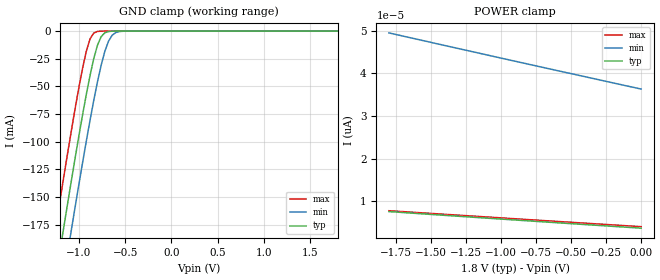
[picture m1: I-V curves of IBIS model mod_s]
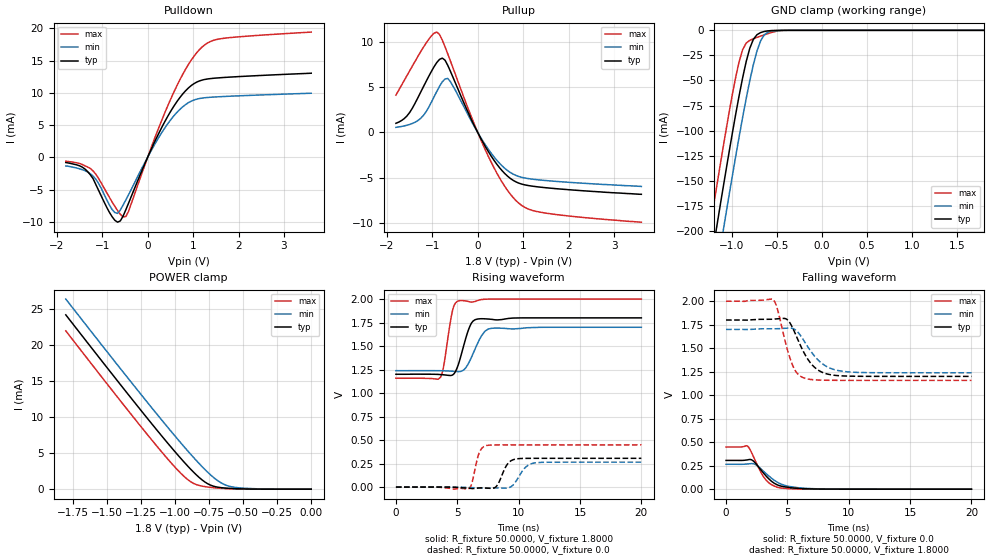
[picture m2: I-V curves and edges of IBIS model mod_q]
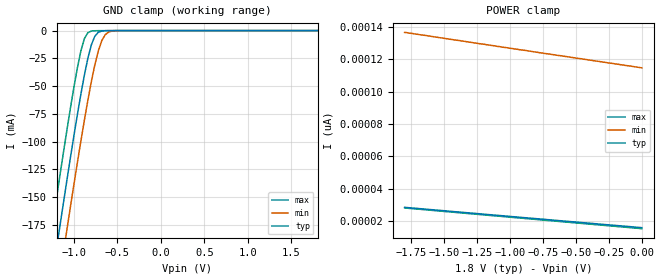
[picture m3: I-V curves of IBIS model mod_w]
| IBIS (I/O, Buffer, Information, Specification) Model, officially
| electronic behavioral standard for Buffer structures of digital pins.
[IBIS ver]  4.0
[File name] m95xxx_c4_tssop8.ibs
[File Rev]  1.0
[Date]   13 May 2016
[Source]   CAD & Design Services (Catania) - STMicroelectronics
[Notes]
   (Note1)  This IBIS model includes the TSSOP8 ceramic package parasitic data
   (Note2)  This IBIS model considers: VCC= 1.80(TYP), 1.70(MIN), 2.00(MAX)
   (Note3)  This IBIS model has some Notes about the non-monotonicity
   of the I-V curves, but they are not indicative of problems
   inside the model;
[Copyright] (c) 2016 STMicroelectronics
|   Component M95XXX
[Component] M95XXX
[Manufacturer] STMicroelectronics
[Package]
| variable   typ   min   max
R_pkg   0.0   0.0   0.0
L_pkg   0.0H   0.0H   0.0H
C_pkg   0.0F   0.0F   0.0F
[Pin]  signal_name   model_name   R_pin   L_pin   C_pin
1   SN   mod_s   NA   NA   NA
2   Q   mod_q   NA   NA   NA
3   WN   mod_w   NA   NA   NA
4   GND   GND   NA   NA   NA
5   D   mod_s   NA   NA   NA
6   C   mod_s   NA   NA   NA
7   HOLDN   mod_h   NA   NA   NA
8   VCCIO   POWER   NA   NA   NA
[Package Model]  182696_TSSOP8
[Define Package Model]  182696_TSSOP8
[Manufacturer]  STMicroelectronics
[OEM]  STMicroelectronics
[Description]  8 pin TSSOP package
[Number Of Pins]  8
[Pin Numbers]
|Pin Num   Terminal Name
1   | net1
2   | net2
3   | net3
4   | net4_GND
5   | net5
6   | net6
7   | net7
8   | net8_VDD
[Model Data]
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[End Model Data]
[End Package Model]
| Models and submodels in the file (4): mod_s (Input), mod_q (I/O), mod_w (Input), mod_h (Input)
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|   Model mod_s
[Model]   mod_s
Model_type Input
Vinl   =   0.540V
Vinh   =   1.260V
C_comp   2.119pF   2.023pF   2.323pF
[Temperature Range]   25.0000   85.0000   -40.0000
[Voltage Range]   1.8000V   1.7000V   2.0000V
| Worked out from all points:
|   GND clamp passes 1 mA (typ) near -0.70 V on its own axis
[GND_clamp]
|Voltage   I(typ)   I(min)   I(max)
-1.8V     -520.5mA   -564.7mA   -476.1mA
-1.28V    -238.3mA   -283.2mA   -192.7mA
-1.24V    -217.2mA   -262.1mA   -171.5mA
-1.16V    -175.3mA   -220.1mA   -129.7mA
-1.08V    -134.2mA   -178.7mA   -89.03mA
-920mV    -57.12mA   -99.32mA   -18.15mA
-840mV    -24.96mA   -62.76mA   -1.769mA
-800mV    -12.85mA   -46.02mA   -321.2uA
-720mV    -1.515mA   -18.31mA   -8.596uA
-680mV    -390.8uA   -9.065mA   -1.39uA
-600mV    -23.11uA   -1.27mA    -36.27nA
1.8V      3.691pA    37.05pA    3.633pA
[POWER_clamp]
|Voltage   I(typ)   I(min)   I(max)
-1.8V     7.58pA     49.51pA    7.783pA
-940mV    5.692pA    43.16pA    5.981pA
-440mV    4.62pA     39.51pA    4.946pA
0V        3.691pA    36.33pA    4.042pA
|   Model mod_q
[Model]   mod_q
Model_type I/O
Polarity   Non-Inverting
Enable   Active-Low
Vinl   =   0.540V
Vinh   =   1.260V
Vmeas  =   0.900V
Cref   =   30pF
C_comp   3.207pF   3.063pF   3.358pF
[Temperature Range]   25.0000   85.0000   -40.0000
[Voltage Range]   1.8000V   1.7000V   2.0000V
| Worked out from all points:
|   slope of the pulldown table from 0 to 0.27 V, typ, clamps not added: 66.3 ohm
|   slope of the pullup table from 0 to 0.27 V, typ, clamps not added: 112 ohm
|   GND clamp passes 1 mA (typ) near -0.63 V on its own axis
|   POWER clamp passes 1 mA (typ) near -0.78 V on its own axis
|   rising waveform, R_fixture 50.0000, V_fixture 1.8000: 20-80 % time 807ps typ, 997ps min, 597ps max; typ from 1.2 V to 1.8 V
|   rising waveform, R_fixture 50.0000, V_fixture 0.0: 20-80 % time 660ps typ, 834ps min, 489ps max; typ from 0 V to 0.306 V
|   falling waveform, R_fixture 50.0000, V_fixture 0.0: 20-80 % time 1.35ns typ, 1.63ns min, 1.13ns max; typ from 0.306 V to 0 V
|   falling waveform, R_fixture 50.0000, V_fixture 1.8000: 20-80 % time 1.48ns typ, 1.68ns min, 1.04ns max; typ from 1.8 V to 1.2 V
[Pulldown]
|Voltage   I(typ)   I(min)   I(max)
-1.8V     -800uA     -1.33mA    -600uA
-1.32V    -2.2mA     -2.27mA    -1.5mA
-1.14V    -4.2mA     -3.38mA    -2.6mA
-720mV    -9.764mA   -8.558mA   -7.616mA
-600mV    -9.857mA   -8.167mA   -8.83mA
-480mV    -8.145mA   -6.616mA   -9.19mA
60mV      953.5uA    798.3uA    1.16mA
420mV     6.082mA    4.991mA    7.619mA
780mV     9.899mA    7.892mA    12.98mA
1.14V     11.86mA    9.13mA     16.72mA
1.62V     12.37mA    9.427mA    18.42mA
3.6V      13.06mA    9.953mA    19.44mA
[Pullup]
|Voltage   I(typ)   I(min)   I(max)
-1.8V     1.015mA    567uA      4.135mA
-1.56V    1.814mA    798uA      6.275mA
-1.26V    4.416mA    1.541mA    8.907mA
-900mV    7.754mA    4.553mA    11.12mA
-780mV    8.236mA    5.606mA    10.23mA
-660mV    7.445mA    5.982mA    8.711mA
-180mV    1.872mA    1.633mA    2.241mA
180mV     -1.666mA   -1.468mA   -2.07mA
540mV     -4.257mA   -3.72mA    -5.541mA
840mV     -5.472mA   -4.759mA   -7.539mA
1.44V     -6.092mA   -5.299mA   -8.888mA
3.6V      -6.85mA    -5.98mA    -9.94mA
[GND_clamp]
|Voltage   I(typ)   I(min)   I(max)
-1.8V     -559.4mA   -602.2mA   -520.2mA
-1.24V    -236.7mA   -280.2mA   -196.2mA
-1.16V    -192mA     -235.6mA   -151.6mA
-1.08V    -148.3mA   -191.6mA   -108.2mA
-960mV    -85.5mA    -127.6mA   -48.31mA
-880mV    -47.65mA   -87.19mA   -19.45mA
-800mV    -17.95mA   -50.29mA   -9.981mA
-760mV    -8.981mA   -34.18mA   -8.395mA
-720mV    -4.357mA   -20.61mA   -7.048mA
-640mV    -1.164mA   -4.638mA   -4.512mA
-520mV    -129.4uA   -370.6uA   -1.197mA
1.8V      87.14pA    20.06nA    65.36pA
[POWER_clamp]
|Voltage   I(typ)   I(min)   I(max)
-1.8V     24.23mA    26.43mA    22mA
-1.42V    15.03mA    17.25mA    12.77mA
-1.14V    8.405mA    10.62mA    6.161mA
-980mV    4.785mA    6.959mA    2.666mA
-920mV    3.503mA    5.631mA    1.558mA
-880mV    2.694mA    4.768mA    984.9uA
-800mV    1.28mA     3.126mA    418.9uA
-740mV    571.4uA    2.017mA    251.7uA
-660mV    208.6uA    867.2uA    116.3uA
-600mV    115.4uA    399.5uA    55.12uA
-380mV    3.21uA     40.27uA    187.1nA
0V        87.14pA    513.3pA    87.73pA
[Ramp]
| variable   typ   min   max
dV/dt_r   0.1836/0.7370n   0.1590/0.9345n   0.2693/0.5509n
dV/dt_f   0.3598/1.5225n   0.2770/1.7831n   0.5057/1.1750n
R_load = 50.0000
[Rising Waveform]
R_fixture= 50.0000
V_fixture= 1.8000
V_fixture_min= 1.7000
V_fixture_max= 2.0000
|time   V(typ)   V(min)   V(max)
0s        1.2V       1.238V     1.158V
3.63ns    1.197V     1.238V     1.167V
3.87ns    1.194V     1.237V     1.272V
4.62ns    1.193V     1.232V     1.88V
5.1ns     1.309V     1.228V     1.98V
5.94ns    1.682V     1.322V     1.972V
6.54ns    1.784V     1.496V     1.978V
7.26ns    1.79V      1.659V     1.999V
7.8ns     1.784V     1.689V     2V
20ns      1.8V       1.7V       2V
[Rising Waveform]
R_fixture= 50.0000
V_fixture= 0.0
V_fixture_min= 0.0
V_fixture_max= 0.0
|time   V(typ)   V(min)   V(max)
0s        3.52nV     39.6nV     3.442nV
5.91ns    -11.9mV    -4.641mV   -21.2mV
6.18ns    -15.05mV   -6.227mV   37.68mV
6.81ns    -9.41mV    -9.347mV   371.1mV
7.41ns    -10.99mV   -12.73mV   442.4mV
8.13ns    184.9uV    -9.096mV   448.3mV
9.09ns    244.5mV    -9.838mV   448.7mV
9.72ns    297.3mV    49.02mV    448.7mV
11.34ns   305.9mV    257.4mV    448.7mV
20ns      306mV      264.8mV    448.7mV
[Falling Waveform]
R_fixture= 50.0000
V_fixture= 0.0
V_fixture_min= 0.0
V_fixture_max= 0.0
|time   V(typ)   V(min)   V(max)
0s        306mV      264.8mV    448.7mV
1.74ns    311.6mV    268mV      459mV
2.205ns   301.7mV    271.1mV    353.7mV
2.745ns   220.5mV    227.4mV    203.7mV
3.135ns   158.9mV    180.6mV    117.4mV
3.585ns   97.74mV    129.3mV    57.86mV
4.305ns   39.42mV    64.97mV    16.15mV
5.205ns   16.62mV    27.67mV    4.807mV
7.185ns   2.061mV    4.824mV    209.2uV
20ns      -6.943nV   55.65nV    -29.02nV
[Falling Waveform]
R_fixture= 50.0000
V_fixture= 1.8000
V_fixture_min= 1.7000
V_fixture_max= 2.0000
|time   V(typ)   V(min)   V(max)
0s        1.8V       1.7V       2V
3.855ns   1.809V     1.707V     2.015V
4.17ns    1.813V     1.707V     1.925V
4.86ns    1.814V     1.712V     1.553V
5.34ns    1.738V     1.713V     1.345V
5.79ns    1.61V      1.679V     1.235V
6.33ns    1.458V     1.583V     1.184V
7.41ns    1.275V     1.386V     1.162V
9.21ns    1.207V     1.26V      1.158V
20ns      1.2V       1.238V     1.158V
|   Model mod_w
[Model]   mod_w
Model_type Input
Vinl   =   0.540V
Vinh   =   1.260V
C_comp   2.119pF   2.023pF   2.323pF
[Temperature Range]   25.0000   85.0000   -40.0000
[Voltage Range]   1.8000V   1.7000V   2.0000V
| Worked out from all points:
|   GND clamp passes 1 mA (typ) near -0.70 V on its own axis
[GND_clamp]
|Voltage   I(typ)   I(min)   I(max)
-1.8V     -520.9mA   -565mA     -476.5mA
-1.28V    -238.6mA   -283.5mA   -193mA
-1.24V    -217.4mA   -262.3mA   -171.8mA
-1.16V    -175.4mA   -220.3mA   -129.9mA
-1.08V    -134.3mA   -178.9mA   -89.23mA
-920mV    -57.23mA   -99.42mA   -18.3mA
-840mV    -25.05mA   -62.84mA   -1.898mA
-800mV    -12.93mA   -46.09mA   -437.7uA
-720mV    -1.573mA   -18.35mA   -100.4uA
-680mV    -437.7uA   -9.105mA   -81.04uA
-600mV    -50.37uA   -1.296mA   -55.9uA
1.8V      15.87pA    115.9pA    13.84pA
[POWER_clamp]
|Voltage   I(typ)   I(min)   I(max)
-1.8V     28.44pA    136.6pA    28.05pA
-1.24V    24.5pA     129.7pA    24.06pA
-1.2V     24.22pA    129.3pA    23.77pA
-1.06V    23.24pA    127.5pA    22.78pA
-880mV    21.99pA    125.4pA    21.5pA
-740mV    21.01pA    123.6pA    20.5pA
-600mV    20.03pA    122pA      19.51pA
-500mV    19.34pA    120.7pA    18.8pA
-460mV    19.06pA    120.3pA    18.52pA
-360mV    18.37pA    119pA      17.81pA
-320mV    18.09pA    118.6pA    17.52pA
0V        15.87pA    114.7pA    15.26pA
